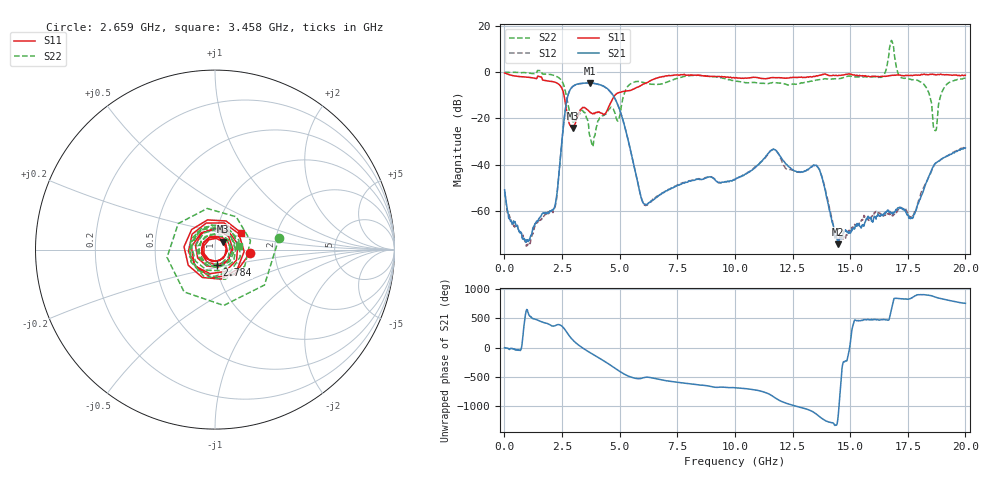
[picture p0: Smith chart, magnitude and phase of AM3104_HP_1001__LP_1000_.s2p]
!Created with skrf (http://scikit-rf.org).
# Hz S RI R 50.0
!freq ReS11 ImS11 ReS21 ImS21 ReS12 ImS12 ReS22 ImS22
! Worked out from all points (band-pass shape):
!   1601 points, 10 MHz to 20 GHz, reference 50 ohm
!   highest |S21| = -4.63 dB at 3.708 GHz (marker M1); lowest = -74.3 dB at 14.48 GHz (marker M2)
!   |S21| within 3 dB of the highest: 2.85 GHz to 4.526 GHz (1.676 GHz wide, 45.4 % of centre)
!   lowest |S11| = -24.1 dB at 2.971 GHz (marker M3), VSWR 1.13, Z = 54.3 + j4.89 ohm
!   |S11| at or under -10 dB: 2.587 GHz to 4.793 GHz (2.206 GHz wide, 59.8 % of centre)
!   |S22| runs from -32.1 to 13.7 dB; largest |S21 - S12| = 0.043
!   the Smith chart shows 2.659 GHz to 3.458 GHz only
!   S11 on the Smith chart (normalised r, x): 2.659 GHz: 1.48, -0.06; 2.784 GHz: 1.01, -0.18; 3.458 GHz: 1.31, +0.26
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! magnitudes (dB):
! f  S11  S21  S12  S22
! 10 MHz  -0.4  -50.8  -51.7  0.0
! 1.022 GHz  -2.2  -73.0  -74.6  -0.4
! 2.109 GHz  -4.1  -59.3  -60.6  -1.2
! 2.659 GHz  -14.2  -15.2  -15.2  -8.8
! 2.784 GHz  -21.2  -9.2  -9.2  -15.1
! 2.971 GHz  -24.1  -6.1  -6.1  -21.4
! 3.346 GHz  -15.8  -4.9  -4.9  -16.7
! 3.458 GHz  -15.3  -4.7  -4.7  -17.4
! 3.708 GHz  -17.2  -4.6  -4.7  -27.6
! 4.883 GHz  -9.2  -13.2  -13.3  -20.6
! 6.032 GHz  -5.2  -56.7  -56.9  -4.5
! 6.682 GHz  -2.3  -53.5  -53.2  -5.3
! 10.01 GHz  -2.5  -46.5  -46.3  -3.9
! 11.64 GHz  -2.4  -33.4  -33.4  -4.5
! 13.34 GHz  -2.1  -40.8  -40.7  -3.9
! 14.48 GHz  -1.5  -74.3  -72.2  -2.8
! 16.68 GHz  -1.6  -60.3  -61.2  7.3
! 17.71 GHz  -1.4  -62.9  -62.1  -3.3
! 18.35 GHz  -1.1  -46.6  -46.7  -7.6
! 18.69 GHz  -1.1  -39.5  -39.5  -25.2
! 19.09 GHz  -1.2  -36.8  -36.8  -6.5
! 20 GHz  -1.4  -32.8  -32.2  -2.6
